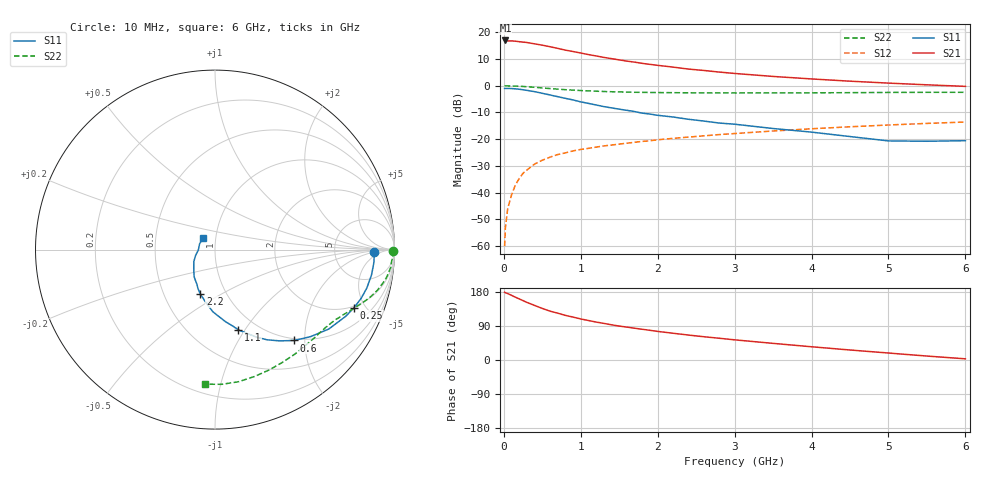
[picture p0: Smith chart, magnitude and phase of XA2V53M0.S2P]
! SIEMENS Discrete & RF Semiconductors
! BFY180
! Si NPN RF Bipolar Junction Transistor in MICRO-X
! VCE = 2.5 V  IC = 3 mA
! Common Emitter S-Parameters:  May  1997
# GHz  S  MA  R  50
!  f  S11  S21  S12  S22
! GHz  MAG  ANG  MAG  ANG  MAG  ANG  MAG  ANG
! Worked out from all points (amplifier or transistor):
!   36 points, 10 MHz to 6 GHz, reference 50 ohm
!   highest |S21| = 16.9 dB at 20 MHz (marker M1)
!   |S21| within 3 dB of that: start of sweep to 706.6 MHz
!   unconditionally stable (mu >= 1): 1.896 GHz to end of sweep
!   at 250 MHz: K = 0.20, MSG = 24.5 dB, |S12| = -32.7 dB
!   at 1.4 GHz: K = 0.87, MSG = 16.2 dB, |S12| = -22.2 dB
!   at 6 GHz: K = 1.09, MAG = 4.8 dB, |S12| = -13.6 dB
!   S11 on the Smith chart (normalised r, x): 10 MHz: 17, -2; 250 MHz: 1.89, -4.14; 600 MHz: 0.96, -1.78; 1.1 GHz: 0.82, -0.94; 2.2 GHz: 0.76, -0.40; 6 GHz: 0.87, +0.12
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0.01  0.8882 -0.8  6.906 178.9  0.001 80.7  0.9922 -0.4
0.02  0.8876 -2.1  7.006 177.7  0.0022 95.4  0.9938 -0.8
0.05  0.8883 -4.6  6.852 175.3  0.005 84.6  0.9918 -1.9
0.1  0.8834 -9.2  6.88 170.6  0.0091 86.8  0.9858 -4.0
0.15  0.8726 -14.2  6.78 165.8  0.0139 81.8  0.9837 -5.8
0.25  0.8389 -22.8  6.523 156.7  0.0231 76.6  0.9668 -9.5
0.3  0.8178 -27.0  6.415 152.0  0.0265 73.8  0.9551 -11.1
0.4  0.7732 -34.9  6.051 144.0  0.0343 69.6  0.9334 -14.0
0.5  0.7205 -42.3  5.718 136.1  0.0405 66.4  0.9075 -16.7
0.6  0.671 -49.0  5.351 128.9  0.0461 63.2  0.8838 -18.9
0.8  0.5803 -60.0  4.619 117.7  0.0555 58.5  0.842 -22.7
1  0.4981 -69.3  4.076 108.3  0.0643 55.2  0.8118 -25.8
1.1  0.4663 -73.7  3.813 104.2  0.0674 53.8  0.799 -27.2
1.3  0.4068 -81.6  3.38 96.6  0.0748 52.0  0.7788 -29.9
1.5  0.3639 -88.5  3.037 89.5  0.0809 50.6  0.764 -32.6
1.9  0.2947 -100.7  2.503 78.3  0.0934 48.2  0.7462 -37.9
2.2  0.2597 -108.5  2.224 70.6  0.1036 46.2  0.74 -41.9
2.8  0.2003 -123.6  1.797 57.4  0.1219 42.7  0.7328 -49.8
3.5  0.1583 -138.4  1.489 43.9  0.1422 38.0  0.7319 -59.1
4.5  0.112 -163.9  1.214 26.4  0.1705 30.7  0.7403 -72.7
5.5  0.0915 159.5  1.038 10.4  0.1972 22.9  0.7515 -87.1
6  0.0937 135.3  0.971 3.1  0.2094 18.6  0.7521 -94.4
